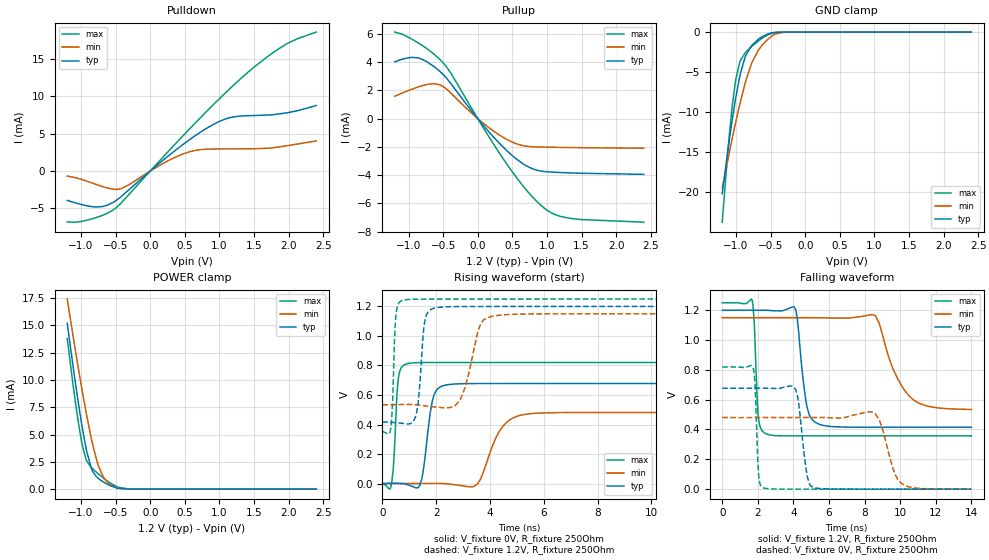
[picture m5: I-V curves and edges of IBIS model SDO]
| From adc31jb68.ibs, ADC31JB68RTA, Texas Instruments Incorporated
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|   Model SDO
[Model]   SDO
Model_type   Output
Polarity   Non-Inverting
Vmeas = 0.6
Vref = 1.2
Cref = 15pF
Rref = 250
|   typ   min   max
|   (nom PVT)   (slow PVT)   (fast PVT)
C_comp   0.281pF   0.233pF   0.342pF
|C_comp High   0.281pF   0.280pF   0.342pF
|C_comp low   0.342pF   0.233pF   0.400pF
[Voltage Range]   1.2   1.15   1.25
[Temperature Range]   27   125   -40
[Pullup Reference]   1.2   1.15   1.25
[Pulldown Reference]   0   0   0
[Power Clamp Reference]   1.2   1.15   1.25
[GND Clamp Reference]   0   0   0
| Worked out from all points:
|   slope of the pulldown table from 0 to 0.18 V, typ, clamps not added: 128 ohm
|   slope of the pullup table from 0 to 0.18 V, typ, clamps not added: 173 ohm
|   GND clamp passes 1 mA (typ) near -0.69 V on its own axis
|   POWER clamp passes 1 mA (typ) near -0.75 V on its own axis
|   falling waveform, V_fixture 1.2V, R_fixture 250Ohm: 20-80 % time 432ps typ, 1.26ns min, 182ps max; typ from 1.2 V to 0.415 V
|   rising waveform, V_fixture 0V, R_fixture 250Ohm: 20-80 % time 283ps typ, 674ps min, 135ps max; typ from 0 V to 0.678 V
|   rising waveform, V_fixture 1.2V, R_fixture 250Ohm: 20-80 % time 189ps typ, 462ps min, 102ps max; typ from 0.416 V to 1.2 V
|   falling waveform, V_fixture 0V, R_fixture 250Ohm: 20-80 % time 381ps typ, 679ps min, 149ps max; typ from 0.676 V to 0 V
[Pulldown]
|   Voltage   I(typ)   I(min)   I(max)
-1.2V     -3.94mA    -679uA     -6.825mA
-793.2mV  -4.818mA   -1.764mA   -6.273mA
-516mV    -4.085mA   -2.451mA   -5.071mA
-300mV    -2.44mA    -1.8mA     -3.071mA
153.6mV   1.202mA    852.3uA    1.55mA
456mV     3.431mA    2.215mA    4.544mA
686.4mV   4.96mA     2.815mA    6.766mA
967.2mV   6.495mA    2.953mA    9.381mA
1.212V    7.257mA    2.969mA    11.55mA
1.788V    7.56mA     3.13mA     15.94mA
1.986V    7.806mA    3.4mA      17.1mA
2.4V      8.771mA    4.03mA     18.6mA
[GND Clamp]
|   Voltage   I(typ)   I(min)   I(max)
-1.2V     -20.18mA   -19.5mA    -23.73mA
-1.124V   -15.16mA   -16.18mA   -15.46mA
-1.096V   -13.35mA   -14.94mA   -12.66mA
-1.056V   -10.98mA   -13.29mA   -9.277mA
-1.006V   -8.231mA   -11.26mA   -5.979mA
-948mV    -5.592mA   -9.069mA   -3.796mA
-868.8mV  -3.121mA   -6.386mA   -2.582mA
-775.2mV  -1.693mA   -3.904mA   -1.807mA
-678mV    -893.1uA   -2.26mA    -1.115mA
-476.4mV  -80.56uA   -450.9uA   -124.2uA
-300mV    -844.5nA   -10.11uA   -1.207uA
2.4V      0A         0A         0A
[Pullup]
|   Voltage   I(typ)   I(min)   I(max)
-1.2V     4.019mA    1.584mA    6.123mA
-872.4mV  4.306mA    2.221mA    5.393mA
-717.6mV  3.965mA    2.429mA    4.887mA
-555.6mV  3.378mA    2.4mA      4.225mA
-390mV    2.488mA    1.817mA    3.225mA
45.6mV    -271.7uA   -189uA     -368.8uA
405.6mV   -2.198mA   -1.434mA   -3.11mA
708mV     -3.354mA   -1.955mA   -5.084mA
960mV     -3.741mA   -2.017mA   -6.327mA
1.111V    -3.796mA   -2.031mA   -6.778mA
1.363V    -3.846mA   -2.049mA   -7.071mA
2.4V      -3.944mA   -2.095mA   -7.329mA
[POWER Clamp]
|   Voltage   I(typ)   I(min)   I(max)
-1.2V     15.2mA     17.42mA    13.8mA
-1.11V    10.99mA    13.81mA    9.275mA
-1.034V   7.697mA    10.9mA     5.926mA
-973.2mV  5.292mA    8.652mA    3.773mA
-930mV    3.82mA     7.145mA    2.779mA
-847.2mV  1.845mA    4.525mA    1.958mA
-753.6mV  992.4uA    2.232mA    1.419mA
-678mV    660.3uA    1.118mA    1.024mA
-584.4mV  341.2uA    437.3uA    588.9uA
-472.8mV  86.99uA    87.72uA    191.6uA
-300mV    1.2uA      2.041uA    2.886uA
2.4V      0A         0A         0A
[Ramp]
R_load = 250
|   typ   min   max
dV/dt_r   0.406798/2.8348e-10   0.288733/6.73939e-10   0.492373/1.34908e-10
dV/dt_f   0.470335/4.32169e-10   0.369097/1.26254e-09   0.535239/1.81555e-10
[Falling Waveform]
V_fixture = 1.2V
V_fixture_min = 1.15V
V_fixture_max = 1.25V
R_fixture = 250Ohm
C_fixture = 0F
|   Time   V(typ)   V(min)   V(max)
0s        1.199V     1.149V     1.249V
1.685ns   1.199V     1.149V     1.265V
2.015ns   1.199V     1.149V     504.2mV
2.382ns   1.199V     1.149V     376.5mV
4.123ns   1.204V     1.15V      357.4mV
4.77ns    548.2mV    1.149V     357.4mV
5.259ns   446.2mV    1.149V     357.4mV
8.6ns     415mV      1.165V     357.2mV
10.52ns   415mV      623mV      357.1mV
14ns      414.9mV    534.2mV    357mV
[Rising Waveform]
V_fixture = 0V
V_fixture_min = 0V
V_fixture_max = 0V
R_fixture = 250Ohm
C_fixture = 0F
|   Time   V(typ)   V(min)   V(max)
0s        -244.4uV   -12.53uV   -353.5uV
319.1ps   1.345mV    -61.47uV   -22.46mV
581.1ps   994.3uV    -101.6uV   689mV
913ps     -6.099mV   49.77uV    811.2mV
1.399ns   -9.309mV   762.4uV    819.4mV
1.866ns   566.1mV    918.6uV    820.1mV
2.257ns   662.6mV    -86.46uV   820.1mV
3.548ns   677.6mV    -510.8uV   820.1mV
5.222ns   677.6mV    466.2mV    820.2mV
14ns      677.8mV    481.2mV    820.3mV
[Rising Waveform]
V_fixture = 1.2V
V_fixture_min = 1.15V
V_fixture_max = 1.25V
R_fixture = 250Ohm
C_fixture = 0F
|   Time   V(typ)   V(min)   V(max)
0s        415.8mV    533.4mV    353.6mV
319.1ps   415.2mV    533.7mV    377.5mV
495.1ps   412.2mV    534.4mV    1.115V
758.9ps   407.9mV    535.3mV    1.241V
1.261ns   463.6mV    533.9mV    1.249V
1.57ns    1.092V     527mV      1.25V
1.866ns   1.185V     520.4mV    1.25V
2.9ns     1.199V     569.1mV    1.25V
3.961ns   1.2V       1.127V     1.25V
14ns      1.2V       1.15V      1.25V
[Falling Waveform]
|Gnd
V_fixture = 0V
V_fixture_min = 0V
V_fixture_max = 0V
R_fixture = 250Ohm
C_fixture = 0F
|   Time   V(typ)   V(min)   V(max)
0s        676.2mV    480.5mV    819.1mV
1.728ns   677mV      479.9mV    814.8mV
1.854ns   677.1mV    479.9mV    675.1mV
2.044ns   677.1mV    480mV      95.72mV
2.314ns   676.8mV    480.1mV    8.829mV
4.123ns   667.5mV    480.5mV    275.4uV
5.049ns   15.83mV    480.4mV    250uV
8.378ns   33.23uV    518.3mV    158.6uV
10.08ns   22.55uV    38.23mV    111.9uV
14ns      -2.157uV   139.1uV    4.09uV
